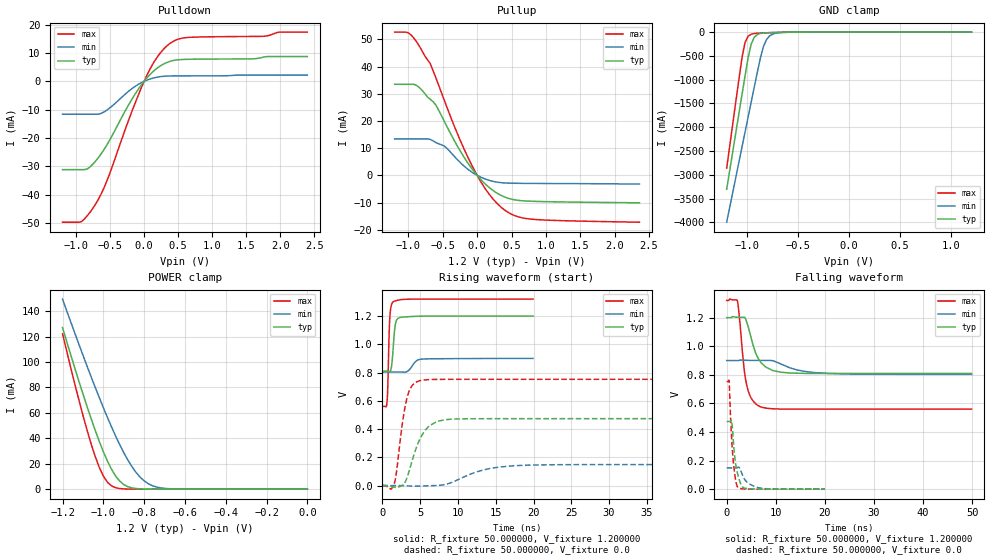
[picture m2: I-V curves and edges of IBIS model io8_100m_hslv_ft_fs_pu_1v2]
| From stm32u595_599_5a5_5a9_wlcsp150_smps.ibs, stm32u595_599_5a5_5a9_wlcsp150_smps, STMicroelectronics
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|   Model io8_100m_hslv_ft_fs_pu_1v2
[Model]  io8_100m_hslv_ft_fs_pu_1v2
Model_type I/O
Polarity   Non-Inverting
Enable   Active-Low
Vinl =   0.360000V
Vinh =   0.840000V
Vmeas =  0.600000V
Cref =   50.000000pF
Rref =   100.000000M
Vref =   0.0V
C_comp   3.030100pF   2.960800pF   3.078300pF
[Temperature Range]   25.000000   0.140000k   -40.000000
[Pullup Reference]   1.200000V   0.900000V   1.320000V
[Pulldown Reference]   0.0V   0.0V   0.0V
[POWER Clamp Reference]   1.200000V   0.900000V   1.320000V
[GND Clamp Reference]   0.0V   0.0V   0.0V
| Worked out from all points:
|   slope of the pulldown table from 0 to 0.18 V, typ, clamps not added: 40.7 ohm
|   slope of the pullup table from 0 to 0.18 V, typ, clamps not added: 39.5 ohm
|   GND clamp passes 1 mA (typ) near -0.51 V on its own axis
|   POWER clamp passes 1 mA (typ) near -0.86 V on its own axis
|   rising waveform, R_fixture 50.000000, V_fixture 1.200000: 20-80 % time 361ps typ, 838ps min, 237ps max; typ from 0.81 V to 1.2 V
|   rising waveform, R_fixture 50.000000, V_fixture 0.0: 20-80 % time 2ns typ, 4.56ns min, 1.18ns max; typ from 0.001 V to 0.474 V
|   falling waveform, R_fixture 50.000000, V_fixture 1.200000: 20-80 % time 2.45ns typ, 5.4ns min, 1.5ns max; typ from 1.2 V to 0.81 V
|   falling waveform, R_fixture 50.000000, V_fixture 0.0: 20-80 % time 1.06ns typ, 2ns min, 809ps max; typ from 0.474 V to 0.001 V
[Pulldown]
|Voltage   I(typ)   I(min)   I(max)
-1.2V     -31.16mA   -11.61mA   -49.71mA
-920mV    -31.16mA   -11.61mA   -49.49mA
-840mV    -31mA      -11.61mA   -47.54mA
-720mV    -28.32mA   -11.61mA   -43.58mA
-560mV    -22.95mA   -10.37mA   -35.89mA
-200mV    -7.146mA   -2.964mA   -11.89mA
0V        0A         0A         0A
160mV     4.047mA    1.298mA    7.361mA
360mV     6.869mA    1.87mA     13mA
640mV     7.765mA    1.923mA    15.46mA
1.76V     8.563mA    2.178mA    15.9mA
2.4V      8.725mA    2.178mA    17.37mA
[Pullup]
|Voltage   I(typ)   I(min)   I(max)
-1.2V     33.49mA    13.42mA    52.69mA
-960mV    33.49mA    13.42mA    51.6mA
-840mV    32.28mA    13.42mA    47.5mA
-680mV    27.89mA    13.19mA    41.04mA
-600mV    25.86mA    12.07mA    35.87mA
-480mV    20.01mA    10.82mA    27.79mA
-280mV    10.44mA    5.592mA    14.93mA
-80mV     2.58mA     1.232mA    3.849mA
160mV     -4.145mA   -1.713mA   -6.415mA
400mV     -7.963mA   -2.792mA   -12.75mA
800mV     -9.537mA   -2.973mA   -16.14mA
2.36V     -10.1mA    -3.2mA     -17.23mA
[GND_clamp]
|Voltage   I(typ)   I(min)   I(max)
-1.2V     -3.305A    -3.998A    -2.862A
-1.05V    -1.316A    -2.418A    -539.3mA
-1.02V    -921mA     -2.103A    -218.8mA
-990mV    -539.5mA   -1.788A    -87.43mA
-960mV    -252.1mA   -1.474A    -44.36mA
-930mV    -110.5mA   -1.16A     -30.32mA
-870mV    -28.03mA   -549.1mA   -21.09mA
-840mV    -18.43mA   -305.6mA   -18.27mA
-810mV    -13.9mA    -159.7mA   -15.73mA
-780mV    -11.23mA   -82.35mA   -13.37mA
-600mV    -2.976mA   -4.272mA   -3.058mA
1.2V      0A         14.73nA    0A
[POWER_clamp]
|Voltage   I(typ)   I(min)   I(max)
-1.2V     127mA      149.4mA    122.2mA
-1.12V    84.98mA    114mA      70.29mA
-1.06V    55.52mA    88.42mA    35.69mA
-1.02V    37.64mA    72.04mA    17.19mA
-1V       29.52mA    64.13mA    10.33mA
-960mV    15.7mA     48.99mA    2.596mA
-900mV    3.636mA    28.77mA    207.8uA
-840mV    502.9uA    13.24mA    43.56uA
-800mV    129uA      6.535mA    43.56uA
-740mV    25.39uA    1.726mA    43.56uA
-620mV    25.22uA    82.33uA    36.06uA
0V        0A         17.33nA    0A
[Ramp]
| variable   typ   min   max
dV/dt_r  0.28389/1.99855n   89.00985m/4.55790n  0.45096/1.18295n
dV/dt_f  0.23433/2.45128n   57.80400m/5.39613n  0.45608/1.50246n
R_load = 50.000000
[Rising Waveform]
R_fixture= 50.000000
V_fixture= 1.200000
V_fixture_min= 0.900000
V_fixture_max= 1.320000
|time   V(typ)   V(min)   V(max)
0s        809.5mV    803.6mV    560mV
600.6ps   810.2mV    803.7mV    581mV
720.7ps   810.1mV    803.7mV    700.8mV
880.9ps   808.6mV    803.7mV    1.048V
1.001ns   807.3mV    803.7mV    1.202V
1.481ns   1.01V      803.7mV    1.302V
1.762ns   1.152V     803.8mV    1.308V
2.402ns   1.191V     803.8mV    1.315V
5.165ns   1.199V     894.8mV    1.32V
19.94ns   1.2V       900mV      1.32V
[Rising Waveform]
R_fixture= 50.000000
V_fixture= 0.0
V_fixture_min= 0.0
V_fixture_max= 0.0
|time   V(typ)   V(min)   V(max)
0s        577.1uV    593.9uV    496.9uV
1.502ns   -9.364mV   559.9uV    945.1uV
1.802ns   -13.72mV   562.4uV    71.35mV
3.203ns   47.25mV    -1.305mV   608.1mV
3.904ns   170mV      -3.121mV   704.6mV
4.905ns   322.2mV    -3.385mV   741.4mV
6.206ns   422.6mV    -640.9uV   750.2mV
9.009ns   469.8mV    19.3mV     752.1mV
17.52ns   473.8mV    141.2mV    752.3mV
49.85ns   473.8mV    149mV      752.3mV
[Falling Waveform]
R_fixture= 50.000000
V_fixture= 1.200000
V_fixture_min= 0.900000
V_fixture_max= 1.320000
|time   V(typ)   V(min)   V(max)
0s        1.2V       900mV      1.32V
2.202ns   1.202V     899.6mV    1.314V
3.504ns   1.202V     902mV      856.2mV
4.104ns   1.166V     901.5mV    723.7mV
5.105ns   1.042V     900.9mV    630.9mV
6.707ns   899.6mV    900.7mV    579.4mV
9.409ns   829.8mV    898.4mV    562.6mV
13.01ns   812.4mV    847.3mV    560.2mV
20.62ns   809.6mV    809.7mV    560mV
49.85ns   809.5mV    803.6mV    560mV
[Falling Waveform]
R_fixture= 50.000000
V_fixture= 0.0
V_fixture_min= 0.0
V_fixture_max= 0.0
|time   V(typ)   V(min)   V(max)
0s        473.8mV    149mV      752.3mV
480.5ps   474mV      149.1mV    758mV
1.001ns   480.2mV    149.1mV    358.7mV
1.281ns   370.6mV    149.1mV    220.5mV
1.642ns   226mV      149mV      105.7mV
1.962ns   150.2mV    149.5mV    38.69mV
2.322ns   94.76mV    153.3mV    11.43mV
3.403ns   11.27mV    84.03mV    2.329mV
6.406ns   1.369mV    11.16mV    630.2uV
19.94ns   577.1uV    593.9uV    496.9uV
